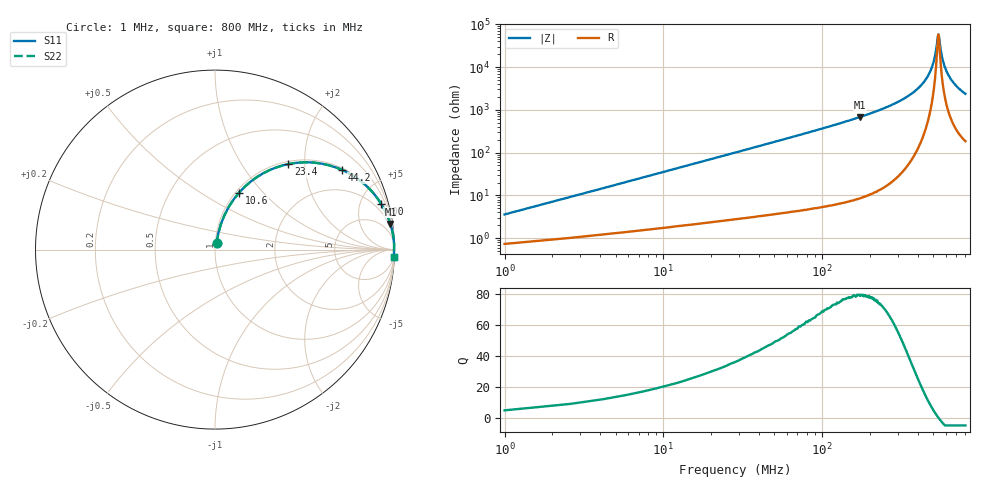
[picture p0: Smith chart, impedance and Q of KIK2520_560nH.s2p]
!version-2
!date-01.2022
!Series
# MHz S RI R 50
!Freq ReS11 ImS11 ReS21 ImS21 ReS12 ImS12 ReS22 ImS22
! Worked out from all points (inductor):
!   501 points, 1 MHz to 800 MHz, reference 50 ohm
!   read as one part in series: L = 560 nH near 4.2 MHz
!   highest Q = 79.6 at 174 MHz (marker M1), where L = 624 nH
!   self-resonance near 540 MHz
!   S11 on the Smith chart (normalised r, x): 1 MHz: 1.01, +0.07; 10.6 MHz: 1.04, +0.75; 23.4 MHz: 1.05, +1.65; 44.2 MHz: 1.07, +3.13; 100 MHz: 1.11, +7.30; 800 MHz: 5, -47
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1  0.0085 0.0346  0.9915 -0.0346  0.9915 -0.0346  0.0085 0.0346
5.8  0.0521 0.1908  0.9479 -0.1908  0.9479 -0.1908  0.0521 0.1908
10.6  0.1339 0.3175  0.8661 -0.3175  0.8661 -0.3175  0.1339 0.3175
15.4  0.2361 0.4058  0.7639 -0.4058  0.7639 -0.4058  0.2361 0.4058
23.4  0.4079 0.4763  0.5921 -0.4763  0.5921 -0.4763  0.4079 0.4763
44.2  0.7063 0.4447  0.2937 -0.4447  0.2937 -0.4447  0.7063 0.4447
66.6  0.8456 0.3526  0.1544 -0.3526  0.1544 -0.3526  0.8456 0.3526
100  0.927 0.2529  0.073 -0.2529  0.073 -0.2529  0.927 0.2529
135  0.9604 0.1885  0.0396 -0.1885  0.0396 -0.1885  0.9604 0.1885
174  0.9772 0.143  0.0228 -0.143  0.0228 -0.143  0.9772 0.143
268  0.9925 0.0792  0.00755 -0.0792  0.00755 -0.0792  0.9925 0.0792
401  0.9977 0.0318  0.00227 -0.0318  0.00227 -0.0318  0.9977 0.0318
451  0.9982 0.0193  0.00176 -0.0193  0.00176 -0.0193  0.9982 0.0193
491  0.9984 0.0103  0.00162 -0.0103  0.00162 -0.0103  0.9984 0.0103
515  0.9984 0.00526  0.00164 -0.00526  0.00164 -0.00526  0.9984 0.00526
534  0.9983 0.00142  0.0017 -0.00142  0.0017 -0.00142  0.9983 0.00142
542  0.9983 -0.000136  0.00173 0.000136  0.00173 0.000136  0.9983 -0.000136
567  0.9981 -0.00496  0.00187 0.00496  0.00187 0.00496  0.9981 -0.00496
591  0.9979 -0.0093  0.00205 0.0093  0.00205 0.0093  0.9979 -0.0093
623  0.9976 -0.0148  0.00236 0.0148  0.00236 0.0148  0.9976 -0.0148
667  0.9971 -0.0219  0.00287 0.0219  0.00287 0.0219  0.9971 -0.0219
800  0.995 -0.0417  0.00503 0.0417  0.00503 0.0417  0.995 -0.0417
